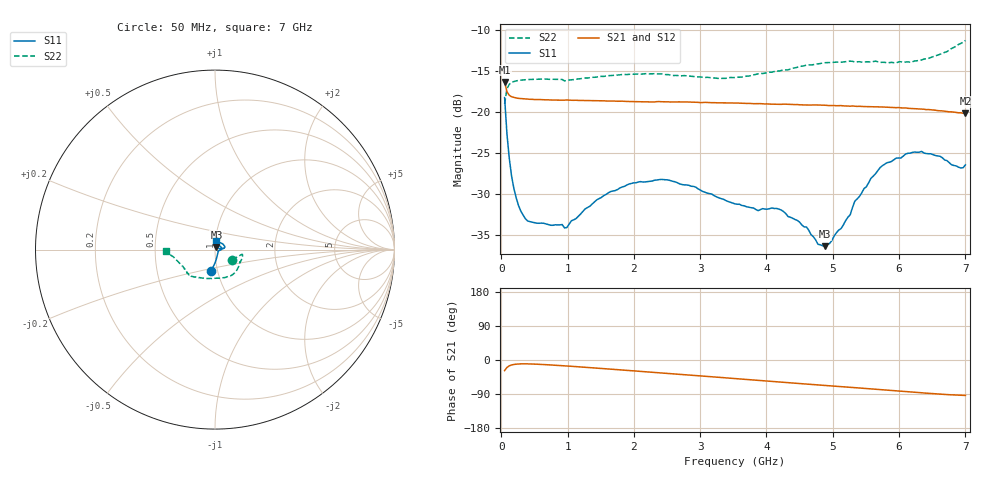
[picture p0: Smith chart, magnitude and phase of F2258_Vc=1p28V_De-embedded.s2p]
! Integrated Device Technology
! Corporate Headquarters
! 6024 Silver Creek Valley Road
! San Jose, CA 95138  USA
! Phone:  1-408-284-8200
! Toll Free:  1-800-223-1366
! Webpage:  http://www.idt.com/
! Timing and RF Division
! 515 Groton Road, Suite 102
! Westford, MA 01886-6024
! Device:  F2258
! Description: Voltage Variable RF Attenuator
! Frequency:  50.0 -  6000.00 MHz
! Package:  3x3 mm Thin QFN Plastic Package: 16 pin
! Ports:  2 RF, 2 DC
!  Pin  1  = NC
!  Pin  2  = NC
!  Pin  3  = RF2  = Port 2
!  Pin  4  = GND
!  Pin  5  = Vdd
!  Pin  6  = NC
!  Pin  7  = VCTRL
!  Pin  8  = NC
!  Pin  9  = GND
!  Pin 10  = RF1  = Port 1
!  Pin 11  = NC
!  Pin 12  = NC
!  Pin 13  = NC
!  Pin 14  = NC
!  Pin 15  = NC
!  Pin 16  = NC
! Vcntrl:  1.280 Volts
! Vdd:  +3.300 Volts
! Current:  1.166 mA
! Data:  The device was measured on a the F2258 evaluation board which has
!  individual transmission lines to the RF pins.  Data was collected
!  using a calibrated network analyzer.  The evaluation board was
!  de-embedded using a TRL calibration technique.
!  The reference plane is the edge of the package pin.
! Misc:  SN 10
!  Action Tracker AT0285
! Date Measured:  2014-12-10
! Date:  2016-01-13  MJV
! Note:
!  Integrated Device Technology supplies this data as a sample of measured
!  data at the package pin for this product.  Your particular data for this
!  product may vary.
!  Data was taken at 25 degrees C.
!  Integrated Device Technology reserves the right to change this data at anytime.
!Freq_(GHz)  S11M_(dB)  S11P_(deg)  S21M_(dB)  S21P_(deg)  S12M_(dB)  S12P_(deg)  S22M_(dB)  S22P_(deg)
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# GHz S dB R 50
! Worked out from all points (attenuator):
!   201 points, 50 MHz to 7 GHz, reference 50 ohm
!   highest |S21| = -16.35 dB at 50 MHz (marker M1); lowest = -20.2 dB at 7 GHz (marker M2)
!   lowest |S11| = -36.4 dB at 4.88 GHz (marker M3), VSWR 1.03, Z = 50.8 + j1.31 ohm
!   |S11| at or under -10 dB: start of sweep to end of sweep
!   |S22| runs from -19.1 to -11.3 dB; largest |S21 - S12| = 0.00089
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0.05  -18.27 -100.0  -16.35 -28.0  -16.35 -27.9  -19.06 -30.6
0.08475  -22.65 -89.7  -17.56 -19.7  -17.56 -19.7  -17.22 -14.9
0.15425  -27.82 -74.9  -18.17 -13.2  -18.13 -13.2  -16.43 -10.4
0.2585  -31.42 -57.2  -18.37 -10.5  -18.32 -10.5  -16.18 -10.2
0.36275  -33.06 -43.6  -18.43 -10.2  -18.42 -10.2  -16.09 -11.9
0.9535  -34.18 -22.4  -18.59 -15.4  -18.54 -15.4  -16.23 -25.9
1.2315  -32.16 -11.4  -18.63 -18.8  -18.58 -18.8  -15.91 -32.7
1.6485  -29.74 -3.5  -18.70 -24.1  -18.65 -24.1  -15.59 -42.1
2.37825  -28.29 13.1  -18.76 -33.6  -18.76 -33.6  -15.38 -58.2
2.8995  -29.12 31.1  -18.83 -40.5  -18.85 -40.5  -15.69 -72.3
3.525  -31.25 64.8  -18.94 -49.0  -18.94 -49.0  -15.82 -95.7
4.22  -32.00 96.7  -19.10 -58.4  -19.07 -58.4  -14.97 -119.2
4.7065  -35.26 80.6  -19.17 -64.8  -19.17 -64.8  -14.25 -129.1
4.88025  -36.42 58.3  -19.21 -67.2  -19.22 -67.1  -14.01 -131.4
5.1235  -34.28 28.1  -19.25 -70.3  -19.25 -70.3  -13.95 -134.5
5.2625  -32.58 15.1  -19.32 -72.1  -19.30 -72.1  -13.82 -136.1
5.332  -30.92 12.1  -19.33 -73.1  -19.32 -73.1  -13.92 -136.5
5.57525  -28.13 7.1  -19.38 -76.2  -19.38 -76.2  -13.93 -140.1
5.85325  -26.17 8.6  -19.46 -80.0  -19.51 -79.8  -14.00 -144.5
6.33975  -24.84 19.2  -19.68 -86.6  -19.69 -86.6  -13.67 -156.8
6.9305  -26.87 72.8  -20.12 -93.1  -20.13 -93.1  -11.66 -175.5
7  -26.49 84.4  -20.21 -93.5  -20.19 -93.6  -11.30 -177.9
